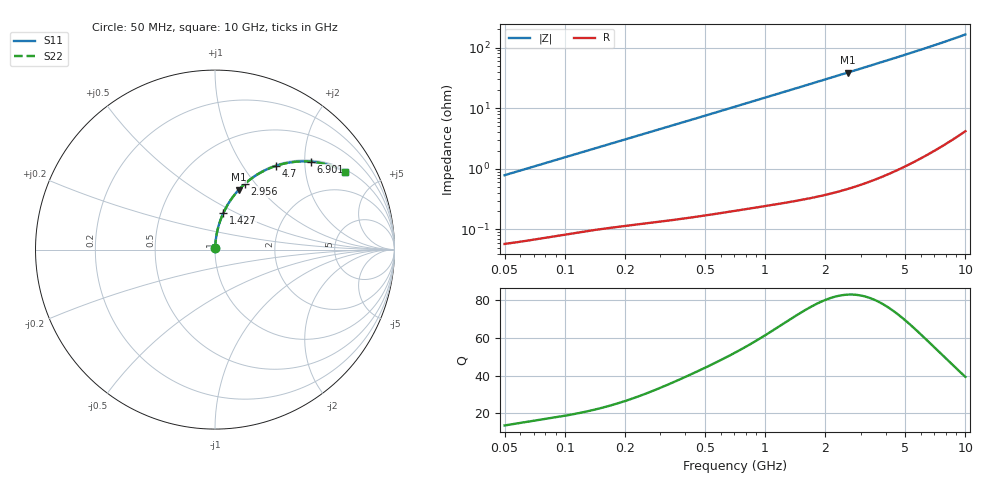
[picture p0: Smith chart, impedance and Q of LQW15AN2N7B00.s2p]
!Murata Part Number: LQW15AN2N7B00
!These Parameters are Measured in Series Mode Connection
!  o--[Z]--o
!Port1  Port2
!  o-------o
!Freq. Start=50[MHz] Stop=10[GHz], 401[Steps]
# Hz S RI R 50
!Freq.(Hz)	S 11(Real)	S 11(Imag)	S 21(Real)	S 21(Imag)	S 12(Real)	S 12(Imag)	S 22(Real)	S 22(Imag)
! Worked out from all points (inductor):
!   401 points, 50 MHz to 10 GHz, reference 50 ohm
!   read as one part in series: L = 2.48 nH near 51.34 MHz
!   highest Q = 83 at 2.59 GHz (marker M1), where L = 2.38 nH
!   S11 on the Smith chart (normalised r, x): 50 MHz: 1.00, +0.02; 1.427 GHz: 1.01, +0.43; 2.956 GHz: 1.01, +0.89; 4.7 GHz: 1.02, +1.43; 6.901 GHz: 1.04, +2.15; 10 GHz: 1.08, +3.28
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5e7  0.000638 0.00782  0.9994 -0.00782  0.9994 -0.00782  0.000638 0.00782
5.134228e7  0.000648 0.00803  0.9994 -0.00803  0.9994 -0.00803  0.000648 0.00803
1.214486e8  0.00126 0.0186  0.9987 -0.0186  0.9987 -0.0186  0.00126 0.0186
1.956524e8  0.00201 0.0296  0.998 -0.0296  0.998 -0.0296  0.00201 0.0296
2.949953e8  0.0033 0.0443  0.9967 -0.0443  0.9967 -0.0443  0.0033 0.0443
4.689809e8  0.00655 0.0698  0.9935 -0.0698  0.9935 -0.0698  0.00655 0.0698
7.071068e8  0.013 0.1042  0.987 -0.1042  0.987 -0.1042  0.013 0.1042
1.011124e9  0.0245 0.1468  0.9755 -0.1468  0.9755 -0.1468  0.0245 0.1468
1.426828e9  0.0459 0.2023  0.9541 -0.2023  0.9541 -0.2023  0.0459 0.2023
1.717543e9  0.0643 0.2388  0.9357 -0.2388  0.9357 -0.2388  0.0643 0.2388
2.122994e9  0.0941 0.2858  0.9059 -0.2858  0.9059 -0.2858  0.0941 0.2858
2.589628e9  0.1333 0.3339  0.8667 -0.3339  0.8667 -0.3339  0.1333 0.3339
2.956399e9  0.1668 0.3668  0.8332 -0.3668  0.8332 -0.3668  0.1668 0.3668
3.511936e9  0.2206 0.4085  0.7794 -0.4085  0.7794 -0.4085  0.2206 0.4085
4.171863e9  0.2865 0.4456  0.7135 -0.4456  0.7135 -0.4456  0.2865 0.4456
4.700058e9  0.3389 0.4664  0.6611 -0.4664  0.6611 -0.4664  0.3389 0.4664
5.733131e9  0.4366 0.4882  0.5634 -0.4882  0.5634 -0.4882  0.4366 0.4882
6.290134e9  0.4852 0.4915  0.5148 -0.4915  0.5148 -0.4915  0.4852 0.4915
6.901252e9  0.5347 0.4899  0.4653 -0.4899  0.4653 -0.4899  0.5347 0.4899
8.198065e9  0.626 0.4736  0.374 -0.4736  0.374 -0.4736  0.626 0.4736
9.738562e9  0.712 0.4407  0.288 -0.4407  0.288 -0.4407  0.712 0.4407
1e10  0.7244 0.4343  0.2756 -0.4343  0.2756 -0.4343  0.7244 0.4343
